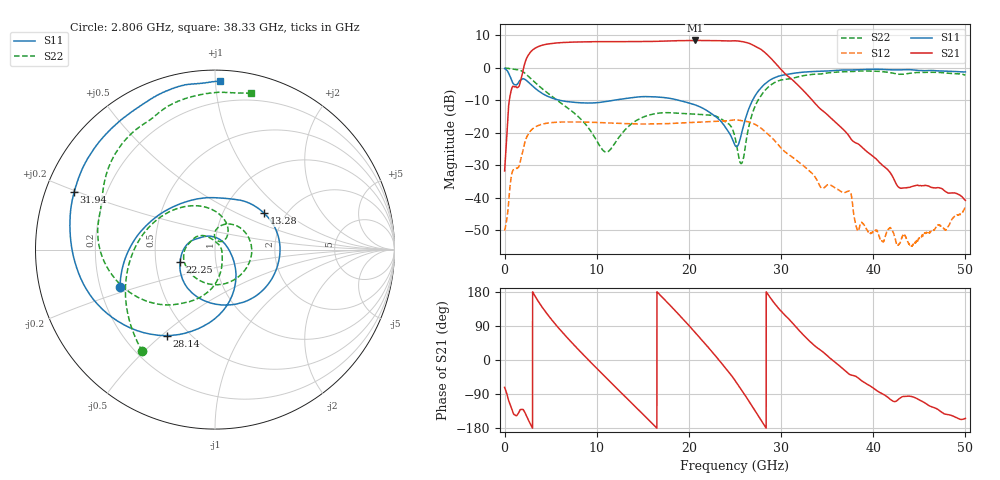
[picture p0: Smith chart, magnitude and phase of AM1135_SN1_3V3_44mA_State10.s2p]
!Agilent Technologies,E8364B,MY43040894,A.07.50.67
!Agilent E8364B: A.07.50.67
!Date: Monday, November 15, 2021 11:11:37
!Correction: S11(Full 2 Port(1,2))
!S21(Full 2 Port(1,2))
!S12(Full 2 Port(1,2))
!S22(Full 2 Port(1,2))
!S2P File: Measurements: S11, S21, S12, S22:
# Hz S  dB  R 50
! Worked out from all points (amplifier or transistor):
!   6401 points, 10 MHz to 50 GHz, reference 50 ohm
!   highest |S21| = 8.5 dB at 20.63 GHz (marker M1)
!   |S21| within 3 dB of that: 3.017 GHz to 27.95 GHz (24.93 GHz wide, 161 % of centre)
!   unconditionally stable (mu >= 1): start of sweep to end of sweep
!   at 8.336 GHz: K = 1.38, MAG = 8.7 dB, |S12| = -16.6 dB
!   at 25 GHz: K = 1.39, MAG = 8.4 dB, |S12| = -16.0 dB
!   at 50 GHz: K = 733.72, MAG = -30.7 dB, |S12| = -42.7 dB
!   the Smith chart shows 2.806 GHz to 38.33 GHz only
!   S11 on the Smith chart (normalised r, x): 2.806 GHz: 0.28, -0.17; 13.28 GHz: 1.56, +0.71; 22.25 GHz: 0.67, -0.10; 28.14 GHz: 0.38, -0.52; 31.94 GHz: 0.09, +0.20; 38.33 GHz: 0.06, +1.03
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1e7  -0.19 -10.5  -31.71 -72.3  -50.08 -49.6  -0.02 -4.6
6.973625e8  -3.21 -60.4  -7.25 -123.0  -34.17 99.8  -0.27 -30.5
2.806316e9  -4.92 -158.6  4.84 -168.9  -19.45 29.2  -3.14 -125.5
3.876414e9  -7.46 165.7  6.81 146.8  -17.48 -15.7  -5.88 -165.0
5.462034e9  -9.56 133.9  7.65 96.0  -16.74 -65.2  -9.42 143.4
8.34427e9  -10.73 95.1  8.02 19.2  -16.64 -137.0  -15.93 66.5
1.04376e10  -10.58 72.6  8.09 -32.7  -16.82 175.8  -24.45 50.0
1.328078e10  -9.35 36.3  8.08 -101.4  -17.14 114.5  -18.45 83.8
1.667854e10  -8.96 -26.0  8.21 176.5  -17.22 42.9  -13.93 14.4
1.892809e10  -9.98 -77.0  8.39 119.5  -16.99 -6.2  -13.96 -45.4
2.063088e10  -11.33 -119.4  8.46 74.1  -16.75 -45.7  -14.21 -96.9
2.224774e10  -13.66 -160.0  8.42 29.3  -16.56 -85.2  -14.53 -145.4
2.359903e10  -16.82 161.7  8.35 -10.0  -16.36 -120.4  -15.86 174.9
2.5005e10  -23.82 75.2  8.36 -53.9  -15.99 -161.6  -21.31 121.3
2.634848e10  -13.75 -55.6  7.75 -102.4  -16.52 153.0  -20.20 -67.2
2.813719e10  -5.19 -119.4  5.02 -170.5  -19.23 88.4  -7.32 -134.8
2.952753e10  -2.73 -157.2  1.04 142.1  -23.06 44.9  -4.18 -173.1
3.194111e10  -1.43 157.8  -5.56 78.5  -29.02 -8.9  -2.67 145.7
3.333927e10  -1.11 138.8  -9.77 44.2  -32.37 -41.9  -2.00 127.1
3.833046e10  -0.55 88.4  -23.33 -46.6  -50.23 -128.3  -0.98 76.9
4.167354e10  -0.55 56.9  -31.61 -100.2  -49.64 -104.6  -1.35 43.7
5e10  -1.22 -63.4  -40.75 -154.1  -42.73 -103.0  -2.23 -68.0
